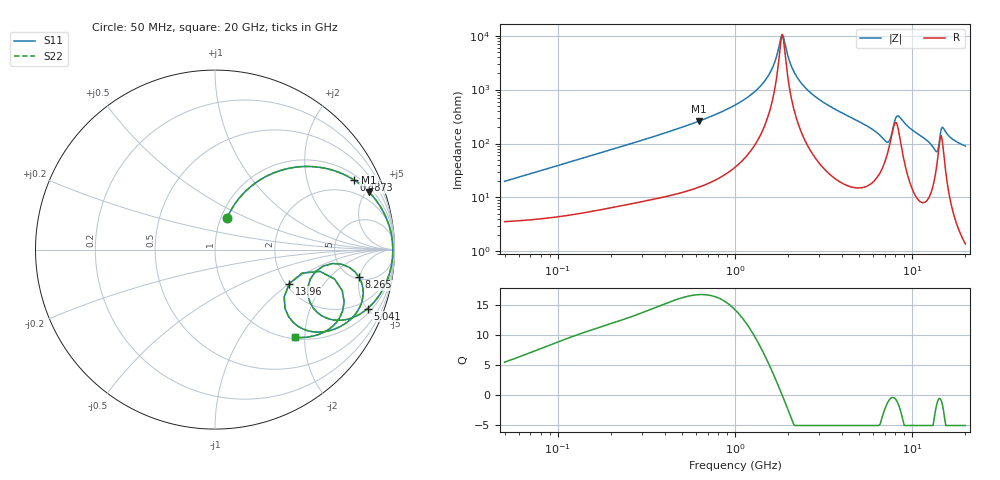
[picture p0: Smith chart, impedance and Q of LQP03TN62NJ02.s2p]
!Murata Part Number: LQP03TN62NJ02
!These Parameters are Measured in Series Mode Connection
!  o--[Z]--o
!Port1  Port2
!  o-------o
!Freq. Start=50[MHz] Stop=20[GHz], 401[Steps]
# Hz S RI R 50
!Freq.(Hz) S11(Real) S11(Imag) S21(Real) S21(Imag) S12(Real) S12(Imag) S22(Real) S22(Imag)
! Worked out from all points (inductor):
!   401 points, 50 MHz to 20 GHz, reference 50 ohm
!   read as one part in series: L = 62.1 nH near 51.52 MHz
!   highest Q = 16.7 at 628.6 MHz (marker M1), where L = 66.1 nH
!   self-resonance near 1.848 GHz
!   S11 on the Smith chart (normalised r, x): 50 MHz: 1.07, +0.39; 487.3 MHz: 1.24, +3.87; 5.041 GHz: 1.30, -5.04; 8.265 GHz: 5.31, -4.91; 13.96 GHz: 2.08, -1.00; 20 GHz: 1.03, -1.79
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5e7  0.0678 0.1765  0.9322 -0.1765  0.9322 -0.1765  0.0678 0.1765
1.364002e8  0.24 0.3813  0.76 -0.3813  0.76 -0.3813  0.24 0.3813
3.721004e8  0.6658 0.4392  0.3342 -0.4392  0.3342 -0.4392  0.6658 0.4392
4.872511e8  0.7756 0.3873  0.2244 -0.3873  0.2244 -0.3873  0.7756 0.3873
6.285508e8  0.8581 0.3203  0.1419 -0.3203  0.1419 -0.3203  0.8581 0.3203
1e9  0.9519 0.1817  0.0481 -0.1817  0.0481 -0.1817  0.9519 0.1817
1.498439e9  0.986 0.0615  0.014 -0.0615  0.014 -0.0615  0.986 0.0615
1.639343e9  0.989 0.0352  0.011 -0.0352  0.011 -0.0352  0.989 0.0352
1.848039e9  0.9906 0.000156  0.00941 -0.000156  0.00941 -0.000156  0.9906 0.000156
2.179053e9  0.9884 -0.0485  0.0116 0.0485  0.0116 0.0485  0.9884 -0.0485
2.728004e9  0.9764 -0.117  0.0236 0.117  0.0236 0.117  0.9764 -0.117
5.041459e9  0.8503 -0.3282  0.1497 0.3282  0.1497 0.3282  0.8503 -0.3282
6.601595e9  0.638 -0.387  0.362 0.387  0.362 0.387  0.638 -0.387
7.442007e9  0.5306 -0.1644  0.4694 0.1644  0.4694 0.1644  0.5306 -0.1644
8.264682e9  0.8027 -0.1535  0.1973 0.1535  0.1973 0.1535  0.8027 -0.1535
9.600142e9  0.7762 -0.3667  0.2238 0.3667  0.2238 0.3667  0.7762 -0.3667
1.166392e10  0.6074 -0.4574  0.3926 0.4574  0.3926 0.4574  0.6074 -0.4574
1.295331e10  0.4632 -0.4277  0.5368 0.4277  0.5368 0.4277  0.4632 -0.4277
1.396067e10  0.4134 -0.1902  0.5866 0.1902  0.5866 0.1902  0.4134 -0.1902
1.460232e10  0.6666 -0.1642  0.3334 0.1642  0.3334 0.1642  0.6666 -0.1642
1.527346e10  0.7115 -0.3411  0.2885 0.3411  0.2885 0.3411  0.7115 -0.3411
2e10  0.447 -0.4896  0.553 0.4896  0.553 0.4896  0.447 -0.4896
